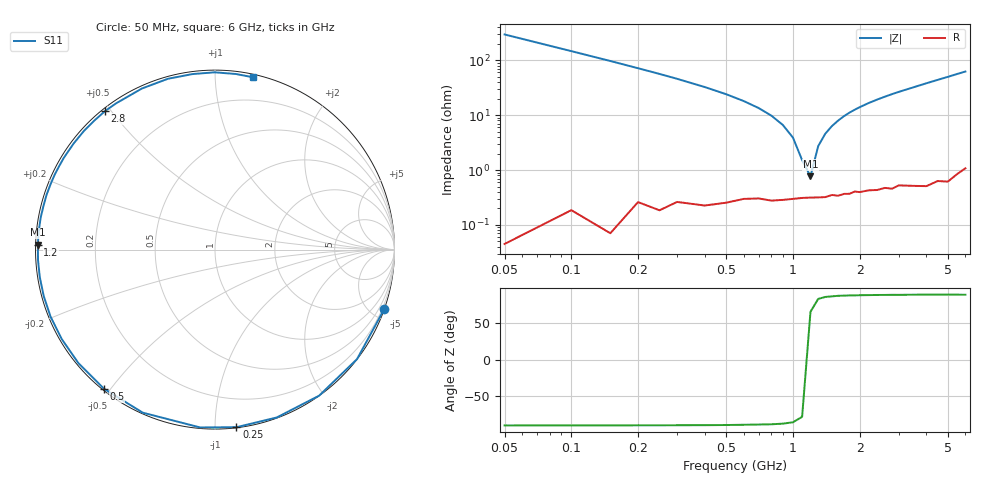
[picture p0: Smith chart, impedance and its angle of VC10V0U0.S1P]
! Infineon Technologies  Discrete & RF Semiconductors
! BBY 56-03
! Si Tuning Diode in SOD323
! VR = 10 V
! S-Parameters:  June  1999
# GHz  S  MA  R  50
!  f  S11
! GHz  MAG  ANG
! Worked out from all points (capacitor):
!   34 points, 50 MHz to 6 GHz, reference 50 ohm
!   read as one part to ground: C = 10.7 pF near 50 MHz
!   lowest |Z| = 766 mohm at 1.2 GHz (marker M1)
!   series resonance near 1.168 GHz, so ESL is about 1.7 nH
!   S11 on the Smith chart (normalised r, x): 50 MHz: 0.00, -5.91; 250 MHz: 0.00, -1.13; 500 MHz: 0.01, -0.48; 1.2 GHz: 0.01, +0.01; 2.8 GHz: 0.01, +0.48; 6 GHz: 0.02, +1.25
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0.05  1 -19.2
0.1  0.9992 -37.6
0.15  0.9994 -54.5
0.2  0.9966 -69.8
0.25  0.9968 -83.1
0.3  0.9943 -94.8
0.4  0.9937 -113.9
0.5  0.9918 -128.6
0.6  0.9895 -140.3
0.7  0.9888 -149.8
0.8  0.9894 -157.9
0.9  0.9888 -164.9
1  0.9882 -171.1
1.2  0.9875 178.4
1.4  0.9873 169.5
1.6  0.9868 161.9
1.8  0.986 154.9
2  0.9854 148.8
2.2  0.9848 143.1
2.4  0.9851 137.9
2.8  0.9853 128.4
3  0.9838 124.1
3.5  0.9856 114.4
4  0.9872 105.4
4.5  0.9859 97.3
5  0.9878 90.1
5.5  0.9853 83.3
6  0.9833 77.4
